|   stm32f427_437_429_439_lqfp144 IBIS Model
[IBIS ver]   4.2
[File name]  stm32f427_437_429_439_lqfp144.ibs
[File Rev]   1.3
[Date]   05-30-2014
[Source] Data Created at STMicroelectronics
[Notes]   File originated from ELDO simulations.
[Disclaimer]  This information is for modeling purpose only and is
   not guaranted. The information is subject to change without
   notice.
[Copyright] Copyright 2014 STMicroelectronics Inc.
[Component] stm32f427_437_429_439_lqfp144
[Manufacturer] STMicroelectronics
[Package]
| variable   typ   min   max
R_pkg   0.0   NA   NA
L_pkg   0.0H   NA   NA
C_pkg   0.0F   NA   NA
[Pin]   signal_name   model_name   R_pin   L_pin   C_pin
1   PE2   io8p_arsudq_ft   1.876E-01   9.420E-09   2.67867E-13
2   PE3   io8p_arsudq_ft   1.824E-01   9.060E-09   2.43844E-13
3   PE4   io8p_arsudq_ft   1.776E-01   8.721E-09   2.21277E-13
4   PE5   io8p_arsudq_ft   1.731E-01   8.405E-09   2.00166E-13
5   PE6   io8p_arsudq_ft   1.689E-01   8.110E-09   1.80511E-13
6   VBAT   POWER   1.650E-01   7.837E-09   1.62311E-13
7   PC13   io8p_arwsudq_ft_v33   1.615E-01   7.586E-09   1.45568E-13
8   PC14   io8p_arwsudq_ft   1.582E-01   7.357E-09   1.30281E-13
9   PC15   io8p_arsudq_ft   1.552E-01   7.150E-09   1.16449E-13
10   PF0   io8p_arsudq_i2cin_ft   1.526E-01   6.964E-09   1.04074E-13
11   PF1   io8p_arsudq_i2cin_ft   1.503E-01   6.801E-09   9.31542E-14
12   PF2   io8p_arsudq_ft   1.482E-01   6.659E-09   8.36906E-14
13   PF3   io8p_arwsudq_ft   1.465E-01   6.539E-09   7.56829E-14
14   PF4   io8p_arwsudq_ft   1.451E-01   6.440E-09   6.91312E-14
15   PF5   io8p_arwsudq_ft   1.441E-01   6.364E-09   6.40354E-14
16   VSS   GND   1.433E-01   6.309E-09   6.03955E-14
17   VDD   POWER   1.428E-01   6.277E-09   5.82116E-14
18   PF6   io8p_arwsudq_ft   1.427E-01   6.266E-09   5.74836E-14
19   PF7   io8p_arwsudq_ft   1.427E-01   6.266E-09   5.74836E-14
20   PF8   io8p_arwsudq_ft   1.428E-01   6.277E-09   5.82116E-14
21   PF9   io8p_arwsudq_ft   1.433E-01   6.309E-09   6.03955E-14
22   PF10   io8p_arwsudq_ft   1.441E-01   6.364E-09   6.40354E-14
23   PH0   io8p_arsudq_ft   1.451E-01   6.440E-09   6.91312E-14
24   PH1   io8p_arsudq_ft   1.465E-01   6.539E-09   7.56829E-14
25   NRST   ioreset_ft_v33   1.482E-01   6.659E-09   8.36906E-14
26   PC0   io8p_ar3wsudq_ft   1.503E-01   6.801E-09   9.31542E-14
27   PC1   io8p_ar3wsudq_ft   1.526E-01   6.964E-09   1.04074E-13
28   PC2   io8p_ar3wsudq_ft   1.552E-01   7.150E-09   1.16449E-13
29   PC3   io8p_ar3wsudq_ft   1.582E-01   7.357E-09   1.30281E-13
30   VDD   POWER   1.615E-01   7.586E-09   1.45568E-13
31   VREFM   POWER   1.650E-01   7.837E-09   1.62311E-13
32   VREFP   POWER   1.689E-01   8.110E-09   1.80511E-13
33   VDDA   POWER   1.731E-01   8.405E-09   2.00166E-13
34   PA0   io8p_ar3wsudq_ft_v33   1.776E-01   8.721E-09   2.21277E-13
35   PA1   io8p_ar3wsudq_ft   1.824E-01   9.060E-09   2.43844E-13
36   PA2   io8p_ar3wsudq_ft   1.876E-01   9.420E-09   2.67867E-13
37   PA3   io8p_ar3wsudq_ft   1.876E-01   9.420E-09   2.67867E-13
38   VSS   GND   1.824E-01   9.060E-09   2.43844E-13
39   VDD   POWER   1.776E-01   8.721E-09   2.21277E-13
40   PA4   io8p_ar3wsudq_ft   1.731E-01   8.405E-09   2.00166E-13
41   PA5   io8p_ar3wsudq_ft   1.689E-01   8.110E-09   1.80511E-13
42   PA6   io8p_ar3wsudq_ft   1.650E-01   7.837E-09   1.62311E-13
43   PA7   io8p_ar3wsudq_ft   1.615E-01   7.586E-09   1.45568E-13
44   PC4   io8p_ar3wsudq_ft   1.582E-01   7.357E-09   1.30281E-13
45   PC5   io8p_ar3wsudq_ft   1.552E-01   7.150E-09   1.16449E-13
46   PB0   io8p_ar3wsudq_ft   1.526E-01   6.964E-09   1.04074E-13
47   PB1   io8p_ar3wsudq_ft   1.503E-01   6.801E-09   9.31542E-14
48   PB2   io8p_ar3wsudq_ft   1.482E-01   6.659E-09   8.36906E-14
49   PF11   io8p_arsudq_ft   1.465E-01   6.539E-09   7.56829E-14
50   PF12   io8p_arsudq_ft   1.451E-01   6.440E-09   6.91312E-14
51   VSS   GND   1.441E-01   6.364E-09   6.40354E-14
52   VDD   POWER   1.433E-01   6.309E-09   6.03955E-14
53   PF13   io8p_arsudq_ft   1.428E-01   6.277E-09   5.82116E-14
54   PF14   io8p_arsudq_ft   1.427E-01   6.266E-09   5.74836E-14
55   PF15   io8p_arsudq_ft   1.427E-01   6.266E-09   5.74836E-14
56   PG0   io8p_arsudq_ft   1.428E-01   6.277E-09   5.82116E-14
57   PG1   io8p_arsudq_ft   1.433E-01   6.309E-09   6.03955E-14
58   PE7   io8p_arsudq_ft   1.441E-01   6.364E-09   6.40354E-14
59   PE8   io8p_arsudq_ft   1.451E-01   6.440E-09   6.91312E-14
60   PE9   io8p_arsudq_ft   1.465E-01   6.539E-09   7.56829E-14
61   VSS   GND   1.482E-01   6.659E-09   8.36906E-14
62   VDD   POWER   1.503E-01   6.801E-09   9.31542E-14
63   PE10   io8p_arsudq_ft   1.526E-01   6.964E-09   1.04074E-13
64   PE11   io8p_arsudq_ft   1.552E-01   7.150E-09   1.16449E-13
65   PE12   io8p_arsudq_ft   1.582E-01   7.357E-09   1.30281E-13
66   PE13   io8p_arsudq_ft   1.615E-01   7.586E-09   1.45568E-13
67   PE14   io8p_arsudq_ft   1.650E-01   7.837E-09   1.62311E-13
68   PE15   io8p_ar3wsudq_ft   1.689E-01   8.110E-09   1.80511E-13
69   PB10   io8p_arsudq_i2cin_ft   1.731E-01   8.405E-09   2.00166E-13
70   PB11   io8p_arsudq_i2cin_ft   1.776E-01   8.721E-09   2.21277E-13
71   VCAP1   POWER   1.824E-01   9.060E-09   2.43844E-13
72   VDD   POWER   1.876E-01   9.420E-09   2.67867E-13
73   PB12   io8usb_id_otg_ft   1.876E-01   9.420E-09   2.67867E-13
74   PB13   io8usb_vbus_otg_ft   1.824E-01   9.060E-09   2.43844E-13
75   PB14   io8usb_lsfs_otg_ft   1.776E-01   8.721E-09   2.21277E-13
76   PB15   io8usb_lsfs_otg_ft   1.731E-01   8.405E-09   2.00166E-13
77   PD8   io8p_arsudq_ft   1.689E-01   8.110E-09   1.80511E-13
78   PD9   io8p_arsudq_ft   1.650E-01   7.837E-09   1.62311E-13
79   PD10   io8p_arsudq_ft   1.615E-01   7.586E-09   1.45568E-13
80   PD11   io8p_arsudq_ft   1.582E-01   7.357E-09   1.30281E-13
81   PD12   io8p_arsudq_ft   1.552E-01   7.150E-09   1.16449E-13
82   PD13   io8p_arsudq_ft   1.526E-01   6.964E-09   1.04074E-13
83   VSS   GND   1.503E-01   6.801E-09   9.31542E-14
84   VDD   POWER   1.482E-01   6.659E-09   8.36906E-14
85   PD14   io8p_arsudq_ft   1.465E-01   6.539E-09   7.56829E-14
86   PD15   io8p_arsudq_ft   1.451E-01   6.440E-09   6.91312E-14
87   PG2   io8p_arsudq_ft   1.441E-01   6.364E-09   6.40354E-14
88   PG3   io8p_arsudq_ft   1.433E-01   6.309E-09   6.03955E-14
89   PG4   io8p_arsudq_ft   1.428E-01   6.277E-09   5.82116E-14
90   PG5   io8p_arsudq_ft   1.427E-01   6.266E-09   5.74836E-14
91   PG6   io8p_arsudq_ft   1.427E-01   6.266E-09   5.74836E-14
92   PG7   io8p_arsudq_ft   1.428E-01   6.277E-09   5.82116E-14
93   PG8   io8p_arsudq_ft   1.433E-01   6.309E-09   6.03955E-14
94   VSS   GND   1.441E-01   6.364E-09   6.40354E-14
95   VDD   POWER   1.451E-01   6.440E-09   6.91312E-14
96   PC6   io8p_arsudq_ft   1.465E-01   6.539E-09   7.56829E-14
97   PC7   io8p_arsudq_ft   1.482E-01   6.659E-09   8.36906E-14
98   PC8   io8p_arsudq_ft   1.503E-01   6.801E-09   9.31542E-14
99   PC9   io8p_arsudq_i2cin_ft   1.526E-01   6.964E-09   1.04074E-13
100   PA8   io8p_arsudq_i2cin_ft   1.552E-01   7.150E-09   1.16449E-13
101   PA9   io8usb_vbus_otg_ft   1.582E-01   7.357E-09   1.30281E-13
102   PA10   io8usb_id_otg_ft   1.615E-01   7.586E-09   1.45568E-13
103   PA11   io8usb_lsfs_otg_ft   1.650E-01   7.837E-09   1.62311E-13
104   PA12   io8usb_lsfs_otg_ft   1.689E-01   8.110E-09   1.80511E-13
105   PA13   io8p_arsudq_ft   1.731E-01   8.405E-09   2.00166E-13
106   VCAP2   POWER   1.776E-01   8.721E-09   2.21277E-13
107   VSS   GND   1.824E-01   9.060E-09   2.43844E-13
108   VDD   POWER   1.876E-01   9.420E-09   2.67867E-13
109   PA14   io8p_arsudq_ft   1.876E-01   9.420E-09   2.67867E-13
110   PA15   io8p_arsudq_ft   1.824E-01   9.060E-09   2.43844E-13
111   PC10   io8p_arsudq_ft   1.776E-01   8.721E-09   2.21277E-13
112   PC11   io8p_arsudq_ft   1.731E-01   8.405E-09   2.00166E-13
113   PC12   io8p_arsudq_ft   1.689E-01   8.110E-09   1.80511E-13
114   PD0   io8p_arsudq_ft   1.650E-01   7.837E-09   1.62311E-13
115   PD1   io8p_arsudq_ft   1.615E-01   7.586E-09   1.45568E-13
116   PD2   io8p_arsudq_ft   1.582E-01   7.357E-09   1.30281E-13
117   PD3   io8p_arsudq_ft   1.552E-01   7.150E-09   1.16449E-13
118   PD4   io8p_arsudq_ft   1.526E-01   6.964E-09   1.04074E-13
119   PD5   io8p_arsudq_ft   1.503E-01   6.801E-09   9.31542E-14
120   VSS   GND   1.482E-01   6.659E-09   8.36906E-14
121   VDD   POWER   1.465E-01   6.539E-09   7.56829E-14
122   PD6   io8p_arsudq_ft   1.451E-01   6.440E-09   6.91312E-14
123   PD7   io8p_arsudq_ft   1.441E-01   6.364E-09   6.40354E-14
124   PG9   io8p_arsudq_ft   1.433E-01   6.309E-09   6.03955E-14
125   PG10   io8p_arsudq_ft   1.428E-01   6.277E-09   5.82116E-14
126   PG11   io8p_arsudq_ft   1.427E-01   6.266E-09   5.74836E-14
127   PG12   io8p_arsudq_ft   1.427E-01   6.266E-09   5.74836E-14
128   PG13   io8p_arsudq_ft   1.428E-01   6.277E-09   5.82116E-14
129   PG14   io8p_arsudq_ft   1.433E-01   6.309E-09   6.03955E-14
130   VSS   GND   1.441E-01   6.364E-09   6.40354E-14
131   VDD   POWER   1.451E-01   6.440E-09   6.91312E-14
132   PG15   io8p_arsudq_ft   1.465E-01   6.539E-09   7.56829E-14
133   PB3   io8p_arsudq_ft   1.482E-01   6.659E-09   8.36906E-14
134   PB4   io8p_arsudq_ft   1.503E-01   6.801E-09   9.31542E-14
135   PB5   io8p_ar3wsudq_ft   1.526E-01   6.964E-09   1.04074E-13
136   PB6   io8p_arsudq_i2cin_ft   1.552E-01   7.150E-09   1.16449E-13
137   PB7   io8p_arsudq_i2cin_ft   1.582E-01   7.357E-09   1.30281E-13
138   BOOT0   vpp_test_hv   1.615E-01   7.586E-09   1.45568E-13
139   PB8   io8p_arsudq_i2cin_ft   1.650E-01   7.837E-09   1.62311E-13
140   PB9   io8p_arsudq_i2cin_ft   1.689E-01   8.110E-09   1.80511E-13
141   PE0   io8p_arsudq_ft   1.731E-01   8.405E-09   2.00166E-13
142   PE1   io8p_arsudq_ft   1.776E-01   8.721E-09   2.21277E-13
143   PDR_ON   io8p_arsudq_ft_v33   1.824E-01   9.060E-09   2.43844E-13
144   VDD   POWER   1.876E-01   9.420E-09   2.67867E-13
[Diff Pin]   inv_pin   vdiff   tdelay_typ  tdelay_min  tdelay_max
75   76   200mV   NA   NA   NA
104   103   200mV   NA   NA   NA
[Model Selector] io8p_ar3wsudq_ft
io8p00_ar3wsudq_ft_pd_lv  "SPEED00 1P8V, PD=40kOhm"
io8p00_ar3wsudq_ft_pu_lv  "SPEED00 1P8V, PU=40kOhm"
io8p00_ar3wsudq_ft_lv  "SPEED00 1P8V"
io8p01_ar3wsudq_ft_pd_lv  "SPEED01 1P8V, PD=40kOhm"
io8p01_ar3wsudq_ft_pu_lv  "SPEED01 1P8V, PU=40kOhm"
io8p01_ar3wsudq_ft_lv  "SPEED01 1P8V"
io8p10_ar3wsudq_ft_pd_lv  "SPEED10 1P8V, PD=40kOhm"
io8p10_ar3wsudq_ft_pu_lv  "SPEED10 1P8V, PU=40kOhm"
io8p10_ar3wsudq_ft_lv  "SPEED10 1P8V"
io8p11_ar3wsudq_ft_pd_lv  "SPEED11 1P8V, PD=40kOhm"
io8p11_ar3wsudq_ft_pu_lv  "SPEED11 1P8V, PU=40kOhm"
io8p11_ar3wsudq_ft_lv  "SPEED11 1P8V"
io8p00_ar3wsudq_ft_pd  "SPEED00, PD=40kOhm"
io8p00_ar3wsudq_ft_pu  "SPEED00, PU=40kOhm"
io8p00_ar3wsudq_ft  "SPEED00"
io8p01_ar3wsudq_ft_pd  "SPEED01, PD=40kOhm"
io8p01_ar3wsudq_ft_pu  "SPEED01, PU=40kOhm"
io8p01_ar3wsudq_ft  "SPEED01"
io8p10_ar3wsudq_ft_pd  "SPEED10, PD=40kOhm"
io8p10_ar3wsudq_ft_pu  "SPEED10, PU=40kOhm"
io8p10_ar3wsudq_ft  "SPEED10"
io8p11_ar3wsudq_ft_pd  "SPEED11, PD=40kOhm"
io8p11_ar3wsudq_ft_pu  "SPEED11, PU=40kOhm"
io8p11_ar3wsudq_ft  "SPEED11"
[Model Selector] io8p_ar3wsudq_ft_v33
io8p00_ar3wsudq_ft_v33_pd_lv  "SPEED00 1P8V, PD=40kOhm"
io8p00_ar3wsudq_ft_v33_pu_lv  "SPEED00 1P8V, PU=40kOhm"
io8p00_ar3wsudq_ft_v33_lv  "SPEED00 1P8V"
io8p01_ar3wsudq_ft_v33_pd_lv  "SPEED01 1P8V, PD=40kOhm"
io8p01_ar3wsudq_ft_v33_pu_lv  "SPEED01 1P8V, PU=40kOhm"
io8p01_ar3wsudq_ft_v33_lv  "SPEED01 1P8V"
io8p10_ar3wsudq_ft_v33_pd_lv  "SPEED10 1P8V, PD=40kOhm"
io8p10_ar3wsudq_ft_v33_pu_lv  "SPEED10 1P8V, PU=40kOhm"
io8p10_ar3wsudq_ft_v33_lv  "SPEED10 1P8V"
io8p11_ar3wsudq_ft_v33_pd_lv  "SPEED11 1P8V, PD=40kOhm"
io8p11_ar3wsudq_ft_v33_pu_lv  "SPEED11 1P8V, PU=40kOhm"
io8p11_ar3wsudq_ft_v33_lv  "SPEED11 1P8V"
io8p00_ar3wsudq_ft_v33_pd  "SPEED00, PD=40kOhm"
io8p00_ar3wsudq_ft_v33_pu  "SPEED00, PU=40kOhm"
io8p00_ar3wsudq_ft_v33  "SPEED00"
io8p01_ar3wsudq_ft_v33_pd  "SPEED01, PD=40kOhm"
io8p01_ar3wsudq_ft_v33_pu  "SPEED01, PU=40kOhm"
io8p01_ar3wsudq_ft_v33  "SPEED01"
io8p10_ar3wsudq_ft_v33_pd  "SPEED10, PD=40kOhm"
io8p10_ar3wsudq_ft_v33_pu  "SPEED10, PU=40kOhm"
io8p10_ar3wsudq_ft_v33  "SPEED10"
io8p11_ar3wsudq_ft_v33_pd  "SPEED11, PD=40kOhm"
io8p11_ar3wsudq_ft_v33_pu  "SPEED11, PU=40kOhm"
io8p11_ar3wsudq_ft_v33  "SPEED11"
[Model Selector] io8p_arsudq_ft
io8p00_arsudq_ft_pd_lv  "SPEED00 1P8V, PD=40kOhm"
io8p00_arsudq_ft_pu_lv  "SPEED00 1P8V, PU=40kOhm"
io8p00_arsudq_ft_lv  "SPEED00 1P8V"
io8p01_arsudq_ft_pd_lv  "SPEED01 1P8V, PD=40kOhm"
io8p01_arsudq_ft_pu_lv  "SPEED01 1P8V, PU=40kOhm"
io8p01_arsudq_ft_lv  "SPEED01 1P8V"
io8p10_arsudq_ft_pd_lv  "SPEED10 1P8V, PD=40kOhm"
io8p10_arsudq_ft_pu_lv  "SPEED10 1P8V, PU=40kOhm"
io8p10_arsudq_ft_lv  "SPEED10 1P8V"
io8p11_arsudq_ft_pd_lv  "SPEED11 1P8V, PD=40kOhm"
io8p11_arsudq_ft_pu_lv  "SPEED11 1P8V, PU=40kOhm"
io8p11_arsudq_ft_lv  "SPEED11 1P8V"
io8p00_arsudq_ft_pd  "SPEED00, PD=40kOhm"
io8p00_arsudq_ft_pu  "SPEED00, PU=40kOhm"
io8p00_arsudq_ft  "SPEED00"
io8p01_arsudq_ft_pd  "SPEED01, PD=40kOhm"
io8p01_arsudq_ft_pu  "SPEED01, PU=40kOhm"
io8p01_arsudq_ft  "SPEED01"
io8p10_arsudq_ft_pd  "SPEED10, PD=40kOhm"
io8p10_arsudq_ft_pu  "SPEED10, PU=40kOhm"
io8p10_arsudq_ft  "SPEED10"
io8p11_arsudq_ft_pd  "SPEED11, PD=40kOhm"
io8p11_arsudq_ft_pu  "SPEED11, PU=40kOhm"
io8p11_arsudq_ft  "SPEED11"
[Model Selector] io8p_arsudq_ft_v33
io8p00_arsudq_ft_v33_pd_lv  "SPEED00 1P8V, PD=40kOhm"
io8p00_arsudq_ft_v33_pu_lv  "SPEED00 1P8V, PU=40kOhm"
io8p00_arsudq_ft_v33_lv  "SPEED00 1P8V"
io8p01_arsudq_ft_v33_pd_lv  "SPEED01 1P8V, PD=40kOhm"
io8p01_arsudq_ft_v33_pu_lv  "SPEED01 1P8V, PU=40kOhm"
io8p01_arsudq_ft_v33_lv  "SPEED01 1P8V"
io8p10_arsudq_ft_v33_pd_lv  "SPEED10 1P8V, PD=40kOhm"
io8p10_arsudq_ft_v33_pu_lv  "SPEED10 1P8V, PU=40kOhm"
io8p10_arsudq_ft_v33_lv  "SPEED10 1P8V"
io8p11_arsudq_ft_v33_pd_lv  "SPEED11 1P8V, PD=40kOhm"
io8p11_arsudq_ft_v33_pu_lv  "SPEED11 1P8V, PU=40kOhm"
io8p11_arsudq_ft_v33_lv  "SPEED11 1P8V"
io8p00_arsudq_ft_v33_pd  "SPEED00, PD=40kOhm"
io8p00_arsudq_ft_v33_pu  "SPEED00, PU=40kOhm"
io8p00_arsudq_ft_v33  "SPEED00"
io8p01_arsudq_ft_v33_pd  "SPEED01, PD=40kOhm"
io8p01_arsudq_ft_v33_pu  "SPEED01, PU=40kOhm"
io8p01_arsudq_ft_v33  "SPEED01"
io8p10_arsudq_ft_v33_pd  "SPEED10, PD=40kOhm"
io8p10_arsudq_ft_v33_pu  "SPEED10, PU=40kOhm"
io8p10_arsudq_ft_v33  "SPEED10"
io8p11_arsudq_ft_v33_pd  "SPEED11, PD=40kOhm"
io8p11_arsudq_ft_v33_pu  "SPEED11, PU=40kOhm"
io8p11_arsudq_ft_v33  "SPEED11"
[Model Selector] io8p_arsudq_i2cin_ft
io8p00_arsudq_i2cin_ft_pd_lv  "SPEED00 1P8V, PD=40kOhm"
io8p00_arsudq_i2cin_ft_pu_lv  "SPEED00 1P8V, PU=40kOhm"
io8p00_arsudq_i2cin_ft_lv  "SPEED00 1P8V"
io8p01_arsudq_i2cin_ft_pd_lv  "SPEED01 1P8V, PD=40kOhm"
io8p01_arsudq_i2cin_ft_pu_lv  "SPEED01 1P8V, PU=40kOhm"
io8p01_arsudq_i2cin_ft_lv  "SPEED01 1P8V"
io8p10_arsudq_i2cin_ft_pd_lv  "SPEED10 1P8V, PD=40kOhm"
io8p10_arsudq_i2cin_ft_pu_lv  "SPEED10 1P8V, PU=40kOhm"
io8p10_arsudq_i2cin_ft_lv  "SPEED10 1P8V"
io8p11_arsudq_i2cin_ft_pd_lv  "SPEED11 1P8V, PD=40kOhm"
io8p11_arsudq_i2cin_ft_pu_lv  "SPEED11 1P8V, PU=40kOhm"
io8p11_arsudq_i2cin_ft_lv  "SPEED11 1P8V"
io8p00_arsudq_i2cin_ft_pd  "SPEED00, PD=40kOhm"
io8p00_arsudq_i2cin_ft_pu  "SPEED00, PU=40kOhm"
io8p00_arsudq_i2cin_ft  "SPEED00"
io8p01_arsudq_i2cin_ft_pd  "SPEED01, PD=40kOhm"
io8p01_arsudq_i2cin_ft_pu  "SPEED01, PU=40kOhm"
io8p01_arsudq_i2cin_ft  "SPEED01"
io8p10_arsudq_i2cin_ft_pd  "SPEED10, PD=40kOhm"
io8p10_arsudq_i2cin_ft_pu  "SPEED10, PU=40kOhm"
io8p10_arsudq_i2cin_ft  "SPEED10"
io8p11_arsudq_i2cin_ft_pd  "SPEED11, PD=40kOhm"
io8p11_arsudq_i2cin_ft_pu  "SPEED11, PU=40kOhm"
io8p11_arsudq_i2cin_ft  "SPEED11"
[Model Selector] io8p_arwsudq_ft
io8p00_arwsudq_ft_pd_lv  "SPEED00 1P8V, PD=40kOhm"
io8p00_arwsudq_ft_pu_lv  "SPEED00 1P8V, PU=40kOhm"
io8p00_arwsudq_ft_lv  "SPEED00 1P8V"
io8p01_arwsudq_ft_pd_lv  "SPEED01 1P8V, PD=40kOhm"
io8p01_arwsudq_ft_pu_lv  "SPEED01 1P8V, PU=40kOhm"
io8p01_arwsudq_ft_lv  "SPEED01 1P8V"
io8p10_arwsudq_ft_pd_lv  "SPEED10 1P8V, PD=40kOhm"
io8p10_arwsudq_ft_pu_lv  "SPEED10 1P8V, PU=40kOhm"
io8p10_arwsudq_ft_lv  "SPEED10 1P8V"
io8p11_arwsudq_ft_pd_lv  "SPEED11 1P8V, PD=40kOhm"
io8p11_arwsudq_ft_pu_lv  "SPEED11 1P8V, PU=40kOhm"
io8p11_arwsudq_ft_lv  "SPEED11 1P8V"
io8p00_arwsudq_ft_pd  "SPEED00, PD=40kOhm"
io8p00_arwsudq_ft_pu  "SPEED00, PU=40kOhm"
io8p00_arwsudq_ft  "SPEED00"
io8p01_arwsudq_ft_pd  "SPEED01, PD=40kOhm"
io8p01_arwsudq_ft_pu  "SPEED01, PU=40kOhm"
io8p01_arwsudq_ft  "SPEED01"
io8p10_arwsudq_ft_pd  "SPEED10, PD=40kOhm"
io8p10_arwsudq_ft_pu  "SPEED10, PU=40kOhm"
io8p10_arwsudq_ft  "SPEED10"
io8p11_arwsudq_ft_pd  "SPEED11, PD=40kOhm"
io8p11_arwsudq_ft_pu  "SPEED11, PU=40kOhm"
io8p11_arwsudq_ft  "SPEED11"
[Model Selector] io8p_arwsudq_ft_v33
io8p00_arwsudq_ft_v33_pd_lv  "SPEED00 1P8V, PD=40kOhm"
io8p00_arwsudq_ft_v33_pu_lv  "SPEED00 1P8V, PU=40kOhm"
io8p00_arwsudq_ft_v33_lv  "SPEED00 1P8V"
io8p01_arwsudq_ft_v33_pd_lv  "SPEED01 1P8V, PD=40kOhm"
io8p01_arwsudq_ft_v33_pu_lv  "SPEED01 1P8V, PU=40kOhm"
io8p01_arwsudq_ft_v33_lv  "SPEED01 1P8V"
io8p10_arwsudq_ft_v33_pd_lv  "SPEED10 1P8V, PD=40kOhm"
io8p10_arwsudq_ft_v33_pu_lv  "SPEED10 1P8V, PU=40kOhm"
io8p10_arwsudq_ft_v33_lv  "SPEED10 1P8V"
io8p11_arwsudq_ft_v33_pd_lv  "SPEED11 1P8V, PD=40kOhm"
io8p11_arwsudq_ft_v33_pu_lv  "SPEED11 1P8V, PU=40kOhm"
io8p11_arwsudq_ft_v33_lv  "SPEED11 1P8V"
io8p00_arwsudq_ft_v33_pd  "SPEED00, PD=40kOhm"
io8p00_arwsudq_ft_v33_pu  "SPEED00, PU=40kOhm"
io8p00_arwsudq_ft_v33  "SPEED00"
io8p01_arwsudq_ft_v33_pd  "SPEED01, PD=40kOhm"
io8p01_arwsudq_ft_v33_pu  "SPEED01, PU=40kOhm"
io8p01_arwsudq_ft_v33  "SPEED01"
io8p10_arwsudq_ft_v33_pd  "SPEED10, PD=40kOhm"
io8p10_arwsudq_ft_v33_pu  "SPEED10, PU=40kOhm"
io8p10_arwsudq_ft_v33  "SPEED10"
io8p11_arwsudq_ft_v33_pd  "SPEED11, PD=40kOhm"
io8p11_arwsudq_ft_v33_pu  "SPEED11, PU=40kOhm"
io8p11_arwsudq_ft_v33  "SPEED11"
[Model Selector] io8usb_id_otg_ft
io8p00_id_otg_ft_pd_lv  "SPEED00 1P8V, PD=14kOhm"
io8p00_id_otg_ft_pu_lv  "SPEED00 1P8V, PU=14kOhm"
io8p00_id_otg_ft_lv  "SPEED00 1P8V"
io8p01_id_otg_ft_pd_lv  "SPEED01 1P8V, PD=14kOhm"
io8p01_id_otg_ft_pu_lv  "SPEED01 1P8V, PU=14kOhm"
io8p01_id_otg_ft_lv  "SPEED01 1P8V"
io8p10_id_otg_ft_pd_lv  "SPEED10 1P8V, PD=14kOhm"
io8p10_id_otg_ft_pu_lv  "SPEED10 1P8V, PU=14kOhm"
io8p10_id_otg_ft_lv  "SPEED10 1P8V"
io8p11_id_otg_ft_pd_lv  "SPEED11 1P8V, PD=14kOhm"
io8p11_id_otg_ft_pu_lv  "SPEED11 1P8V, PU=14kOhm"
io8p11_id_otg_ft_lv  "SPEED11 1P8V"
io8p00_id_otg_ft_pd  "SPEED00, PD=14kOhm"
io8p00_id_otg_ft_pu  "SPEED00, PU=14kOhm"
io8p00_id_otg_ft  "SPEED00"
io8p01_id_otg_ft_pd  "SPEED01, PD=14kOhm"
io8p01_id_otg_ft_pu  "SPEED01, PU=14kOhm"
io8p01_id_otg_ft  "SPEED01"
io8p10_id_otg_ft_pd  "SPEED10, PD=14kOhm"
io8p10_id_otg_ft_pu  "SPEED10, PU=14kOhm"
io8p10_id_otg_ft  "SPEED10"
io8p11_id_otg_ft_pd  "SPEED11, PD=14kOhm"
io8p11_id_otg_ft_pu  "SPEED11, PU=14kOhm"
io8p11_id_otg_ft  "SPEED11"
[Model Selector] io8usb_lsfs_otg_ft
io8usb_ls_otg_ft_dpdn_pd  "LS USB DP/DN IO + PD=20kOhm"
io8usb_ls_otg_ft_dpdn_pupu2  "LS USB DP/DN IO + PU/PU2=2.2kOhm"
io8usb_ls_otg_ft_dpdn_pu2  "LS USB DP/DN IO + PU2=1.2kOhm"
io8usb_ls_otg_ft_dpdn_pu  "LS USB DP/DN IO + PU=1.2kOhm"
io8usb_ls_otg_ft_dpdn  "LS USB DP/DN IO"
io8usb_fs_otg_ft_dpdn_pd  "HS USB DP/DN IO + PD=20kOhm"
io8usb_fs_otg_ft_dpdn_pupu2  "HS USB DP/DN IO + PU/PU2=2.2kOhm"
io8usb_fs_otg_ft_dpdn_pu2  "HS USB DP/DN IO + PU2=1.2kOhm"
io8usb_fs_otg_ft_dpdn_pu  "HS USB DP/DN IO + PU=1.2kOhm"
io8usb_fs_otg_ft_dpdn  "HS USB DP/DN IO"
io8p00_lsfs_otg_ft_pd_lv  "SPEED00 1P8V, PD=40kOhm"
io8p00_lsfs_otg_ft_pu_lv  "SPEED00 1P8V, PU=40kOhm"
io8p00_lsfs_otg_ft_lv  "SPEED00 1P8V"
io8p01_lsfs_otg_ft_pd_lv  "SPEED01 1P8V, PD=40kOhm"
io8p01_lsfs_otg_ft_pu_lv  "SPEED01 1P8V, PU=40kOhm"
io8p01_lsfs_otg_ft_lv  "SPEED01 1P8V"
io8p10_lsfs_otg_ft_pd_lv  "SPEED10 1P8V, PD=40kOhm"
io8p10_lsfs_otg_ft_pu_lv  "SPEED10 1P8V, PU=40kOhm"
io8p10_lsfs_otg_ft_lv  "SPEED10 1P8V"
io8p11_lsfs_otg_ft_pd_lv  "SPEED11 1P8V, PD=40kOhm"
io8p11_lsfs_otg_ft_pu_lv  "SPEED11 1P8V, PU=40kOhm"
io8p11_lsfs_otg_ft_lv  "SPEED11 1P8V"
io8p00_lsfs_otg_ft_pd  "SPEED00, PD=40kOhm"
io8p00_lsfs_otg_ft_pu  "SPEED00, PU=40kOhm"
io8p00_lsfs_otg_ft  "SPEED00"
io8p01_lsfs_otg_ft_pd  "SPEED01, PD=40kOhm"
io8p01_lsfs_otg_ft_pu  "SPEED01, PU=40kOhm"
io8p01_lsfs_otg_ft  "SPEED01"
io8p10_lsfs_otg_ft_pd  "SPEED10, PD=40kOhm"
io8p10_lsfs_otg_ft_pu  "SPEED10, PU=40kOhm"
io8p10_lsfs_otg_ft  "SPEED10"
io8p11_lsfs_otg_ft_pd  "SPEED11, PD=40kOhm"
io8p11_lsfs_otg_ft_pu  "SPEED11, PU=40kOhm"
io8p11_lsfs_otg_ft  "SPEED11"
[Model Selector] io8usb_vbus_otg_ft
io8psenb_vbus_otg_ft  "VBUS PULSE, SENSE VB"
io8psenab_vbus_otg_ft  "VBUS PULSE, SENSE VA and VB"
io8psena_vbus_otg_ft  "VBUS PULSE, SENSE VA"
io8psen_vbus_otg_ft  "VBUS PULSE"
io8p00_vbus_otg_ft_pd_lv  "SPEED00 1P8V, PD=40kOhm"
io8p00_vbus_otg_ft_pu_lv  "SPEED00 1P8V, PU=40kOhm"
io8p00_vbus_otg_ft_lv  "SPEED00 1P8V"
io8p01_vbus_otg_ft_pd_lv  "SPEED01 1P8V, PD=40kOhm"
io8p01_vbus_otg_ft_pu_lv  "SPEED01 1P8V, PU=40kOhm"
io8p01_vbus_otg_ft_lv  "SPEED01 1P8V"
io8p10_vbus_otg_ft_pd_lv  "SPEED10 1P8V, PD=40kOhm"
io8p10_vbus_otg_ft_pu_lv  "SPEED10 1P8V, PU=40kOhm"
io8p10_vbus_otg_ft_lv  "SPEED10 1P8V"
io8p11_vbus_otg_ft_pd_lv  "SPEED11 1P8V, PD=40kOhm"
io8p11_vbus_otg_ft_pu_lv  "SPEED11 1P8V, PU=40kOhm"
io8p11_vbus_otg_ft_lv  "SPEED11 1P8V"
io8p00_vbus_otg_ft_pd  "SPEED00, PD=40kOhm"
io8p00_vbus_otg_ft_pu  "SPEED00, PU=40kOhm"
io8p00_vbus_otg_ft  "SPEED00"
io8p01_vbus_otg_ft_pd  "SPEED01, PD=40kOhm"
io8p01_vbus_otg_ft_pu  "SPEED01, PU=40kOhm"
io8p01_vbus_otg_ft  "SPEED01"
io8p10_vbus_otg_ft_pd  "SPEED10, PD=40kOhm"
io8p10_vbus_otg_ft_pu  "SPEED10, PU=40kOhm"
io8p10_vbus_otg_ft  "SPEED10"
io8p11_vbus_otg_ft_pd  "SPEED11, PD=40kOhm"
io8p11_vbus_otg_ft_pu  "SPEED11, PU=40kOhm"
io8p11_vbus_otg_ft  "SPEED11"
[Model Selector] ioreset_ft_v33
ioreset_ft_v33_pu_lv  "ioreset 1P8V + PU=40kOhm"
ioreset_ft_v33_nopu_lv  "ioreset 1P8V"
ioreset_ft_v33_pu  "ioreset + PU=40kOhm"
ioreset_ft_v33_nopu  "ioreset"
[Model Selector] vpp_test_hv
vpp_test_hv_2p4  "Input Buffer 1P8V"
vpp_test_hv_3p3  "Input Buffer"
| Models and submodels in the file (260): io8p00_ar3wsudq_ft_pd_lv (I/O), io8p00_ar3wsudq_ft_pu_lv (I/O), io8p00_ar3wsudq_ft_lv (I/O), io8p01_ar3wsudq_ft_pd_lv (I/O), io8p01_ar3wsudq_ft_pu_lv (I/O), io8p01_ar3wsudq_ft_lv (I/O), io8p10_ar3wsudq_ft_pd_lv (I/O), io8p10_ar3wsudq_ft_pu_lv (I/O), io8p10_ar3wsudq_ft_lv (I/O), io8p11_ar3wsudq_ft_pd_lv (I/O), io8p11_ar3wsudq_ft_pu_lv (I/O), io8p11_ar3wsudq_ft_lv (I/O), io8p00_ar3wsudq_ft_pd (I/O), io8p00_ar3wsudq_ft_pu (I/O), io8p00_ar3wsudq_ft (I/O), io8p01_ar3wsudq_ft_pd (I/O), io8p01_ar3wsudq_ft_pu (I/O), io8p01_ar3wsudq_ft (I/O), io8p10_ar3wsudq_ft_pd (I/O), io8p10_ar3wsudq_ft_pu (I/O), io8p10_ar3wsudq_ft (I/O), io8p11_ar3wsudq_ft_pd (I/O), io8p11_ar3wsudq_ft_pu (I/O), io8p11_ar3wsudq_ft (I/O), io8p00_ar3wsudq_ft_v33_pd_lv (I/O), io8p00_ar3wsudq_ft_v33_pu_lv (I/O), io8p00_ar3wsudq_ft_v33_lv (I/O), io8p01_ar3wsudq_ft_v33_pd_lv (I/O), io8p01_ar3wsudq_ft_v33_pu_lv (I/O), io8p01_ar3wsudq_ft_v33_lv (I/O), io8p10_ar3wsudq_ft_v33_pd_lv (I/O), io8p10_ar3wsudq_ft_v33_pu_lv (I/O), io8p10_ar3wsudq_ft_v33_lv (I/O), io8p11_ar3wsudq_ft_v33_pd_lv (I/O), io8p11_ar3wsudq_ft_v33_pu_lv (I/O), io8p11_ar3wsudq_ft_v33_lv (I/O), io8p00_ar3wsudq_ft_v33_pd (I/O), io8p00_ar3wsudq_ft_v33_pu (I/O), io8p00_ar3wsudq_ft_v33 (I/O), io8p01_ar3wsudq_ft_v33_pd (I/O), io8p01_ar3wsudq_ft_v33_pu (I/O), io8p01_ar3wsudq_ft_v33 (I/O), io8p10_ar3wsudq_ft_v33_pd (I/O), io8p10_ar3wsudq_ft_v33_pu (I/O), io8p10_ar3wsudq_ft_v33 (I/O), io8p11_ar3wsudq_ft_v33_pd (I/O), io8p11_ar3wsudq_ft_v33_pu (I/O), io8p11_ar3wsudq_ft_v33 (I/O), io8p00_arsudq_ft_pd_lv (I/O), io8p00_arsudq_ft_pu_lv (I/O), io8p00_arsudq_ft_lv (I/O), io8p01_arsudq_ft_pd_lv (I/O), io8p01_arsudq_ft_pu_lv (I/O), io8p01_arsudq_ft_lv (I/O), io8p10_arsudq_ft_pd_lv (I/O), io8p10_arsudq_ft_pu_lv (I/O), io8p10_arsudq_ft_lv (I/O), io8p11_arsudq_ft_pd_lv (I/O), io8p11_arsudq_ft_pu_lv (I/O), io8p11_arsudq_ft_lv (I/O), io8p00_arsudq_ft_pd (I/O), io8p00_arsudq_ft_pu (I/O), io8p00_arsudq_ft (I/O), io8p01_arsudq_ft_pd (I/O), io8p01_arsudq_ft_pu (I/O), io8p01_arsudq_ft (I/O), io8p10_arsudq_ft_pd (I/O), io8p10_arsudq_ft_pu (I/O), io8p10_arsudq_ft (I/O), io8p11_arsudq_ft_pd (I/O), io8p11_arsudq_ft_pu (I/O), io8p11_arsudq_ft (I/O), io8p00_arsudq_ft_v33_pd_lv (I/O), io8p00_arsudq_ft_v33_pu_lv (I/O), io8p00_arsudq_ft_v33_lv (I/O), io8p01_arsudq_ft_v33_pd_lv (I/O), io8p01_arsudq_ft_v33_pu_lv (I/O), io8p01_arsudq_ft_v33_lv (I/O), io8p10_arsudq_ft_v33_pd_lv (I/O), io8p10_arsudq_ft_v33_pu_lv (I/O)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
